FUNCTION_BLOCK FB_SFP_EGU_EGK_IO_Link_Cyclic_Protocol

   VAR_INPUT 
	  	  	
	  b_RELEASE_FUNKTION_BLOCK : BOOL; 
      b_00_FAST_STOP : BOOL;
      b_01_STOP : Bool;
      b_02_ACKNOLEDGE : Bool;
      b_03_PREPARE_FOR_SHUTDOWN : Bool;
      b_04_SOFTRESET : Bool;
      b_05_RELEASE_FOR_MANUAL_MOVEMENT : BOOL;
      b_06_REPEAT_COMMAND_TOGGLE : Bool;
      b_07_GRIP_DIREKTION : BOOL;
	  
      b_08_JOG_MODE_NEGATIVE : Bool;
      b_09_JOG_MODE_POSITIVE : Bool;
      b_11_RELEASE_WORKPIECE : BOOL;
      b_12_GRIP_WORKPIECE : Bool;
      b_13_MOVE_TO_ABSOLUTE_POS : Bool;
      b_14_MOVE_TO_RELATIVE_POS : Bool;
      b_16_GRIP_WORKPIECE_AT_EXPECTED_POSITION : BOOL;
	  b_31_GRIP_FORCE_AND_POSITION_MAINTAINANCE_ACTIVATED : BOOL; 
      di_POSSITIONING : DInt;
      di_VELOCITY : DInt;
      di_GRIPPING_FORCE : DINT;
	  
	  dw_STATUS_DWORD_GRIPPER : DWORD;
	  di_IN_ACTUAL_POSITION : DINT;
	  dw_IN_DIAGNOSE : DWORD;
   END_VAR

   VAR_OUTPUT 
	  
      b_00_READY_FOR_OPPERATION : Bool;
      b_01_CONTOL_AUTHORITY_FIELDBUS : Bool;
      b_02_READY_FOR_SHUTDOWN : Bool;
      b_03_NOT_FEASIBLE : Bool;
      b_04_COMMAND_SUCCESSFULLY_PROCESSED : Bool;
      b_05_COMMAND_RECEIVED_TOGGLE : Bool;
      b_06_WARNING : Bool;
      b_07_ERROR : Bool;
      b_08_BRAKE_RELEASD : Bool;
      b_09_SOFTWARELIMIT_REACHED : Bool;
      b_10_REFERENCED : Bool;
      b_11_NO_WORKPIECE_DETECTED : Bool;
      b_12_WORKPIECE_GRIPPED : Bool;
      b_13_POSITION_REACHED : Bool;
      b_14_WORKPIECE_PRE_GRIPPED_STARTED : Bool;
      b_16_WORKPIECE_LOST : Bool;
      b_17_WRONG_WORKPIECE_DETECTED : BOOL;
	  b_31_ACTIVATE_GRIP_FORCE_AND_POSITION_MAINTAINANCE : BOOL;
	  di_ACTUAL_POSITION : DINT;
      i_DIAGNOSE_WARNUNG : Word;
      i_DIAGNOSE_ERROR : WORD;
	  
	  dw_CONTROL_DW_GRIPPER : DWORD;
	  di_OUT_POSSITIONING : DINT;
	  di_OUT_VELOCITY : DINT;
	  di_OUT_GRIPPING_FORCE : DINT;
	  
   END_VAR
   
   
   VAR_TEMP 
      b_Temp_OUT_15 : BOOL;
	  b_Temp_OUT_18 : BOOL;
	  b_Temp_OUT_19 : BOOL;
	  b_Temp_OUT_20 : BOOL;
	  b_Temp_OUT_21 : BOOL;
	  b_Temp_OUT_22 : BOOL;
	  b_Temp_OUT_23 : BOOL;
	  b_Temp_OUT_24 : BOOL;
	  b_Temp_OUT_25 : BOOL;
	  b_Temp_OUT_26 : BOOL;
	  b_Temp_OUT_27 : BOOL;
	  b_Temp_OUT_28 : BOOL;
	  b_Temp_OUT_29 : BOOL;
	  b_Temp_OUT_30 : BOOL;
	  
	  b_Temp_IN_1 : BOOL;
	  b_Temp_in_2 : BOOL;
	  b_Temp_in_3 : BOOL;
	  b_Temp_in_4 : BOOL;
	  b_Temp_in_5 : BOOL;
	  b_Temp_in_6 : BOOL;
	  b_Temp_in_7 : BOOL;
	  b_Temp_in_8 : BOOL;
	  b_Temp_in_9 : BOOL;
	  b_Temp_in_10 : BOOL;
	  b_Temp_in_11 : BOOL;
	  b_Temp_in_12 : BOOL;
	  b_Temp_in_13 : BOOL;
	  b_Temp_in_14 : BOOL;
	  b_Temp_in_15 : BOOL;
	  b_Temp_in_16 : BOOL;
	  b_Temp_in_17 : BOOL;
	  b_Temp_in_18 : BOOL;
	  b_Temp_in_19 : BOOL;
	  b_Temp_in_20 : BOOL;
	  b_Temp_in_21 : BOOL;
	  b_Temp_in_22 : BOOL;
	  b_Temp_in_23 : BOOL;
	  b_Temp_in_24 : BOOL;
	  b_Temp_in_25 : BOOL;
	  b_Temp_in_26 : BOOL;
	  b_Temp_in_27 : BOOL;
	  b_Temp_in_28 : BOOL;
	  b_Temp_in_29 : BOOL;
	  b_Temp_in_30 : BOOL;
	  b_Temp_in_31 : BOOL;
	  	  
   END_VAR
(*
   VAR 
	  TYPE Input:
	  STRUCT 
      //Input : Struct
         dw_Status_DW : DWord;
         di_Actual_Position : DInt;
         di_Reserved_byte_4_to_byte_7 : DInt;
         i_Diagnostic_Warning : Word;
         i_Diagnostic_Error : Word;
      END_STRUCT
	  END_TYPE
		  
      TYPE Status_DW:
		  STRUCT
         b_Ready_For_Operation : BOOL;
         b_Control_Authority : Bool;
         b_Ready_For_Shutdown : Bool;
         b_Not_Feasible : Bool;
         b_Success : Bool;
         b_Command_Received_Toggle : Bool;
         b_Warning : Bool;
         b_Error : Bool;
         b_Brake_released : Bool;
         b_Sofwarelimit : Bool;
         b_Referenced : Bool;
         b_No_Workpiece_Detected : Bool;
         b_Gripped : Bool;
         b_Position_Reached : Bool;
         b_Pre_Gripped : Bool;
         b_Reserved_1_6 : Bool;
         b_Workpiece_Lost : Bool;
         b_Wrong_Workpiece_Detected : Bool;
         b_Reserved_2_2 : Bool;
         b_Reserved_2_3 : Bool;
         b_Reserved_2_4 : Bool;
         b_Reserved_2_5 : Bool;
         b_Reserved_2_6 : Bool;
         b_Reserved_2_7 : Bool;
         b_Reserved_3_0 : Bool;
         b_Reserved_3_1 : Bool;
         b_Reserved_3_2 : Bool;
         b_Reserved_3_3 : Bool;
         b_Reserved_3_4 : Bool;
         b_Reserved_3_5 : Bool;
         b_Reserved_3_6 : Bool;
         b_Reserved_3_7 : Bool;
      END_STRUCT
	  END_TYPE
	  
	  TYPE Output:
		  STRUCT
         dw_Steuerwort : DWord;
         di_Position : DInt;
         di_Velocity : DInt;
         di_Gripping_Force : DInt;
      END_STRUCT
	  END_TYPE
	  
	  Control_DW: STRUCT;
		  
	  END_STRUCT
      TYPE Control_DW:
		STRUCT 
         b_Fast_Stop : Bool;
         b_Stop : Bool;
         b_Acknoledge : Bool;
         b_Prerare_For_Shutdown : Bool;
         b_Softreset : Bool;
         b_Release_Brake : Bool;
         b_Repeat_Command_Toggle : Bool;
         b_Grip_Direction : Bool;
         b_Jog_Mode_Negative : Bool;
         b_Jog_Mode_Positive : Bool;
         b_Reference : Bool;
         b_Release_Workpiece : Bool;
         b_Grip_Workpiece : Bool;
         b_Move_To_Absolute_Position : Bool;
         b_Move_To_Relative_Position : Bool;
         b_Reserved_1_7 : Bool;
         b_Grip_Workpiece_With_Expected_Position : Bool;
         b_Reserved_2_1 : Bool;
         b_Reserved_2_2 : Bool;
         b_Reserved_2_3 : Bool;
         b_Reserved_2_4 : Bool;
         b_Reserved_2_5 : Bool;
         b_Reserved_2_6 : Bool;
         b_Reserved_2_7 : Bool;
         b_Reserved_3_0 : Bool;
         b_Reserved_3_1 : Bool;
         b_Reserved_3_2 : Bool;
         b_Reserved_3_3 : Bool;
         b_Reserved_3_4 : Bool;
         b_Reserved_3_5 : Bool;
         b_Reserved_3_6 : Bool;
         b_Reserved_3_7 : Bool;
      END_STRUCT
	  END_TYPE
      //GETIO_Instance {InstructionName := 'GETIO'; LibVersion := '1.1'} : GETIO;
      //SETIO_Instance {InstructionName := 'SETIO'; LibVersion := '1.2'} : SETIO;
   END_VAR

   VAR_TEMP 
      reserved_ed_8 : DInt;
   END_VAR

*)



	(*
	FUNCTION_BLOCK FB_SFP_Zyclic_Protokol
	TITLE = 'FB_SFP_EGU_EGK_IO_Link_Cyclic_Protocol'
	VERSION : '1.0.1'
	AUTHOR  : 'SCHUNK'
	NAME    : 'FB_Zyklische_Kommunikation_SFP_Beckhoff TwinCAT 3'
	FAMILY  : 'SCHUNK'
	Projekt Nr.:
	=============================================================================
	 Schunk GmbH&Co.KG
	 (c)Copyright (2022) All Rights Reserved
	-----------------------------------------------------------------------------
	 Library:       Schunk
	 Tested with:   TWINCAT 3 Build 4024.32
	 Engineering:   TWINCAT 3 Build 4024.32
	 Restrictions:  XXX(OB types, etc.)
	 Requirements:  (hardware, technological package, memory needed, etc.)
	 Functionality: The Funktion Block communicates Cyclic with the Gripper to read and Wright Data
	  
	*************************************************************************
	Historie
	####################
	1.0.1
	- Bugfix Input Bit 31
	
	####################
	1.0.0
	Release Funktion Block
	
	
	*************************************************************************)
	
	//MANUAL ENGLISH 
	    
	    // Statement section REGION
	    
	    (*************************************************************************    
	    The function block is TO read AND transfer cyclic parameters that are changed FOR specific functions in the device
	    can be used TO make The application process safer OR faster.
	    
	    Input parameters:
	    ------------------
	    b_RELEASE_FUNKTION_BLOCK		: Release FOR processing the block
	    
	    b_00_FAST_STOP					: immediate shutdown OF The process currently running in The gripper AND shutdown OF The motor phases
	    b_01_STOP						: Pausing AND stopping the currently running process.
	    b_02_ACKNOLEDGE 				: Acknowledge fault
	    b_03_PREPARE_FOR_SHUTDOWN		: Initiate the restoration OF data on The device in preparation FOR switching off OR rebooting
	    b_04_SOFTRESET					: Warm start OF The device
	    b_05_RELEASE_FOR_MANUAL_MOVEMENT: The brake can be released FOR 5 seconds in the "ERROR_FAST_STOP" state
	    b_06_REPEAT_COMMAND_TOGGLE		: The command that is still pending can, IF it is a repeatable command, be repeated without loss OF Time FOR each positive AND negative change OF this bit
	    b_07_GRIP_DIRECTION				: determines The gripping direction. FALSE = external gripping (the workpiece is gripped from the outside) / True = internal gripping (the workpiece is gripped from the inside).
	    
	    b_08_JOG_MODE_NEGATIVE			: Simple movement OF The device in negative direction. Function also possible without "REFERENCE".
	    b_09_JOG_MODE_POSITIVE			: Simple movement OF The device in The positive direction. Function also possible without "REFERENCE".
	    b_10_Reserved					: 
	    b_11_RELEASE_WORKPIECE			: IF The status is "GRIPPED", the gripper is opened in the opposite direction AND the workpiece is released
	    b_12_GRIP_WORKPIECE				: the gripper executes a movement that should lead TO gripping a workpiece. Internal speed parameters are used here
	    b_13_MOVE_TO_ABSOLUTE_POSITION	: The gripper jaws are moved TO The position specified in The cyclic protocol at The specified speed.
	    b_14_MOVE_TO_RELATIVE_POSITION	: The gripper jaws are moved TO The calculated position with The position specified in The cyclic protocol at The specified speed.
	    b_15_Reserved					: 
		
	    b_16_GRIP_WORKPIECE_AT_EXPECTED_POSITION : the gripper performs a movement which is intended to grip a workpiece. Here, the position value is assumed as the workpiece size. Due to the workpiece size, it is pre-positioned accordingly and then gripped. See software manual for more information.
		b_17_Reserved					: 
		b_18_Reserved					: 
		b_19_Reserved					: 
		b_20_Reserved					: 
		b_21_Reserved					: 
		b_22_Reserved					: 
		b_23_Reserved					: 
		
		b_24_Reserved					: 
		b_25_Reserved					: 
		b_26_Reserved					: 
		b_27_Reserved					: 
		b_28_Reserved					: 
		b_29_Reserved					: 
		b_30_Reserved					: 
		b_31_ACTIVATE_GRIP_FORCE_AND_POSITION_MAINTAINANCE	: Maintaining the gripping force by locking the gripper jaws with a brake.
	    
		dw_STATUS_DWORD_GRIPPER 		: Input double word of the gripper which comes from the hardware and is split into individual bits in the block
		di_IN_ACTUAL_POSITION 			: Current position of the gripper. Is only passed on to the output parameter of the block.
		dw_IN_DIAGNOSE 					: Diagnostic double word of the gripper. Is split into warning and error in the block.
		
	    #################
	    
	    Output parameters:
	    ------------------
	    
	    b_00_READY_FOR_OPPERATION		:   indicates that the gripper is ready FOR operation
	    b_01_CONTOL_AUTHORITY_FIELDBUS  :   indicates whether the fieldbus has control authority over the gripper
	    b_02_READY_FOR_SHUTDOWN			:   signals readiness FOR shutdown OR restart after the request "Prepare for shutdown"
	    b_03_NOT_FEASIBLE				:	Indicates that the last issued command cannot be executed.
	    									Possible causes are:
	        								- a new command was sent although the command that is still active has NOT yet been processed.
	        								- 2 OR more control commands simultaneously active in the control word
	        								- Parameter data FOR position, speed OR force are outside the permissible limits.
	    
	    b_04_COMMAND_SUCCESSFULLY_PROCESSED	: indicates that the last executable command was successfully processed.
	    b_05_COMMAND_RECEIVED_TOGGLE		: Indicates that a command was sent TO The gripper via The bus. the command does NOT have TO be processed OR started at the time it is displayed.
	    b_06_WARNING						: signals a warning in the gripper, e.g. temperature warning
	    b_07_ERROR							: signals a fault in the gripper, e.g. rapid stop
		
	    b_08_BRAKE_RELEASD					: Signals that the brake is released IF a brake is installed in The gripper.
	    b_09_SOFTWARELIMIT_REACHED			: indicates that the gripper has reached a software limit
	    b_10_REFERENCED						: indicates that the gripper is referenced
	    b_11_NO_WORKPIECE_DETECTED			: indicates that no workpiece was detected
	    b_12_WORKPIECE_GRIPPED				: signals that a workpiece has been gripped
	    b_13_POSITION_REACHED				: signals that the relative OR absolute position has been approached
	    b_14_WORKPIECE_PRE_GRIPPED_STARTED  : indicates that the gripper has started the pre-gripping function
		b_15_Reserved						: 
		
	    b_16_WORKPIECE_LOST					: signals that the gripped workpiece was lost
	    b_17_WRONG_WORKPIECE_DETECTED		: signals that a wrong workpiece was detected
		b_18_RESERVED						: 
		b_19_RESERVED						: 
		b_20_RESERVED						: 
		b_21_RESERVED						: 
		b_22_RESERVED						: 
		b_23_RESERVED						: 
		
		b_24_RESERVED						: 
		b_25_RESERVED						: 
		b_26_RESERVED						: 
		b_27_RESERVED						: 
		b_28_RESERVED						: 
		b_29_RESERVED						: 
		b_30_RESERVED						: 
		b_31_GRIP_FORCE_AND_POSITION_MAINTAINANCE_ACTIVATED : Maintaining the gripping force by locking the gripper jaws with a brake is active.
		
	    di_ACTUAL_POSITION					: the current position OF The gripper is returned here
	    i_DIAGNOSE_WARNUNG					: Output of the gripper's warning code
	    i_DIAGNOSE_ERROR					: Output of the error code of the gripper
	        
	    *************************************************************************)
	    
// MANUAL GERMAN
	    
	(*************************************************************************
	    Der Baustein soll Zyklische Parameter einlesen und übertragen, welche für bestimmte Funktionen im Gerät geändert 
	    werden können um den Applikationsprozess sicherer oder schneller zu machen.
	    
	    Eingangsparameter:
	    ------------------
	    
	    b_RELEASE_FUNKTION_BLOCK : Freigabe zur Bearbeitung des Bausteins
	    
	    b_00_FAST_STOP					: sofortiges Abschalten des aktuell im Greifer laufenden Prozesses und abschalten der Motorphasen
	    b_01_STOP						: Anhalten und Stoppen des Aktuell laufenden Prozesses.
	    b_02_ACKNOLEDGE					: Störung Quittieren
	    b_03_PREPARE_FOR_SHUTDOWN		: Anstoßen der Rückspeicherung von Daten auf dem Grät un Vorbereitung zum Ausschalten oder Reboot
	    b_04_SOFTRESET					: Warmstart des Gerätes
	    b_05_RELEASE_FOR_MANUAL_MOVEMENT: Lösen der Bremse für 5 Sekunden im Zustand "ERROR_FAST_STOP" möglich
	    b_06_REPEAT_COMMAND_TOGGLE		: Das Noch anstehende Kommando kann, sofern es ein wiederholbares Kommando ist, ohne zeitverlust bei jedem positiven und negativen wechsel dieses Bits wiederholt werden 
	    b_07_GRIP_DIRECTION				: legt die Greifrichtung fest. FALSE = Ausengreifen (Das Werkstück wird von ausen gegriffen) / True = Innengreifen (Das Werkstück wird von innen gegriffen). 
	    
	    b_08_JOG_MODE_NEGATIVE			: einfaches Verfahren des Gerätes in negative Richtung. Funktion auch ohne Referenz möglich.
	    b_09_JOG_MODE_POSITIVE			: einfaches Verfahren des Gerätes in positive Richtung. Funktion auch ohne Referenz möglich.
	    b_10_RESERVED					: Referenzieren des Gerätes wird angestoßen
	    b_11_RELEASE_WORKPIECE			: Bei Status "GRIPPED" wird der Greifer in die entgegegesetzte Richtung geöffnet und das Werkstück freigegeben
	    b_12_GRIP_WORKPIECE				: der Greifer führt eine Bewegung aus, welche zum greifen eines Werkstückes führen soll. Hierbei werden interne Geschwindigkeitsparameter genommen
	    b_13_MOVE_TO_ABSOLUTE_POSITION	: Die Greiferbacken werden auf die im Zyklischen Protokoll vorgegebene Position mit der vorgegebenen Geschwindigkeit gefahren. 
	    b_14_MOVE_TO_RELATIVE_POSITION	: Die Greiferbacken werden auf die errechnete Position mit der im Zyklischen Protokoll vorgegebene Position mit der vorgegebenen Geschwindigkeit gefahren.
	    b_15_Reserved					: 
		
	    b_16_GRIP_WORKPIECE_AT_EXPECTED_POSITION : der Greifer führt eine Bewegung aus, welche zum greifen eines Werkstückes führen soll. Hirbei wird der Positionswert als Werkstückgröße angenommen. aufgrund der Werkstückgröße wird entsprechend Vorpositioniert und dann gegriffen. Weitere Informationen siehe Softwarehandbuch.
		b_17_Reserved					: 
		b_18_Reserved					: 
		b_19_Reserved					: 
		b_20_Reserved					: 
		b_21_Reserved					: 
		b_22_Reserved					: 
		b_23_Reserved					: 
		
		b_24_Reserved					: 
		b_25_Reserved					: 
		b_26_Reserved					: 
		b_27_Reserved					: 
		b_28_Reserved					: 
		b_29_Reserved					: 
		b_30_Reserved					: 
		b_31_ACTIVATE_GRIP_FORCE_AND_POSITION_MAINTAINANCE	: Erhaltung der Greifkraft durch festsetzen der Greifbackendurch eine Bremse.
              

		dw_STATUS_DWORD_GRIPPER 		: Eingangsdoppelwort des Greifers welches von der Hardware kommt und im Baustein in einzelbits aufgesplittet wird
		di_IN_ACTUAL_POSITION 			: Aktuelle Position des Greifers. Wird nur durchgereicht auf den Ausgangsparameter des Bausteins.
		dw_IN_DIAGNOSE 					: Diagnosedoppelwort des Greifers. Wird im Baustein zu Warning und Error aufgesplittet.
            
	    ##################    
    
	    Ausgangsparameter:
	    ------------------
	    
	    b_00_READY_FOR_OPPERATION			: zeigt die Betriebsbereitschaft des Greifers an
	    b_01_CONTOL_AUTHORITY_FIELDBUS		: zeigt an, ob der Feldbus die Steuerhoheit über den Greifer hat
	    b_02_READY_FOR_SHUTDOWN				: signalisiert die Bereitschaft zum Abschalten bzw Neustarten nach der Anforderung "Prepare for shutdown"
	    b_03_NOT_FEASIBLE					: Zeigt an, das der zuletzt abgesetzte Befehl nicht ausgeführt werden kann.
	                            				Mögliche Ursachen sind:
	                                			- ein neuer Befehl wurde abgesetzt, obwohl der noch aktive Befehl noch nicht abgearbeitet wurde.
	                                			- 2 oder mehr Steuerbefehle gleichzeitig aktiv im Steuerwort
	                                			- Parameterdaten von Position, Geschwindigkeit oder Kraft liegen auserhalb der Zulässigen grenzen. 
	                                
	    b_04_COMMAND_SUCCESSFULLY_PROCESSED	: zeigt das erfolgreiche Abarbeiten des letzten ausführbaren Befehls an.
	    b_05_COMMAND_RECEIVED_TOGGLE		: Zeigt an, das ein Befehl über den Bus an den Greufer gesendet wurde. zum Zeitpunkt der Anzeige muß der Befehl noch nicht abgearbeitet oder gestartet sein.
	    b_06_WARNING						: signalisiert eine Warnung im Greifer, z.B. Temperaturwarnung
	    b_07_ERROR							: signalisiert eine Störung im Greifer, z.B. Schnellstop
		
	    b_08_BRAKE_RELEASD					: Signalisiert, dass die Bremse geöffnet ist, sofern eine Bremse im Greifer verbaut ist.
	    b_09_SOFTWARELIMIT_REACHED			: signalisiert, das der Greifer eine Softwarelimit angefahren hat
	    b_10_REFERENCED						: signalisiert, das der Greifer referenziert ist 
	    b_11_NO_WORKPIECE_DETECTED			: signalisiert, dass kein Werkstück erkannt wurde
	    b_12_WORKPIECE_GRIPPED				: signalisiert, dass ein Werkstück gegriffen wurde
	    b_13_POSITION_REACHED				: signalisiert, dass die relative oder absolute Possition angefahren wurde
	    b_14_WORKPIECE_PRE_GRIPPED_STARTED  : signalisiert, dass der Greifer die Pre Gripping Funktion angestoßen hat
		b_15_RESERVED						: 
		
	    b_16_WORKPIECE_LOST					: signalisiert, dass das gegriffene Werkstück verloren ging
	    b_17_WRONG_WORKPIECE_DETECTED		: signalisiert, das ein falsches Werkstück erkannt wurde
		b_18_RESERVED						: 
		b_19_RESERVED						: 
		b_20_RESERVED						: 
		b_21_RESERVED						: 
		b_22_RESERVED						: 
		b_23_RESERVED						: 
		
		b_24_RESERVED						: 
		b_25_RESERVED						: 
		b_26_RESERVED						: 
		b_27_RESERVED						: 
		b_28_RESERVED						: 
		b_29_RESERVED						: 
		b_30_RESERVED						: 
		b_31_GRIP_FORCE_AND_POSITION_MAINTAINANCE_ACTIVATED : Erhaltung der Greifkraft durch festsetzen der Greifbackendurch eine Bremse ist aktiv.
				
	    di_ACTUAL_POSITION					: hier wird die aktuelle Possition des Greifers zurückgegeben
	    i_DIAGNOSE_WARNUNG					: Ausgabe des Warnungscodes des Greifers
	    i_DIAGNOSE_ERROR					: Ausgabe des Störungscodes des Greifers
	    
	*************************************************************************)
	    
	// Release FB
	    // Statement section REGION
	    		
	    IF  
				b_RELEASE_FUNKTION_BLOCK = TRUE
	    THEN
	       
			b_00_READY_FOR_OPPERATION 			:= DW_STATUS_DWORD_GRIPPER.0;
			b_01_CONTOL_AUTHORITY_FIELDBUS 		:= DW_STATUS_DWORD_GRIPPER.1;
			b_02_READY_FOR_SHUTDOWN 			:= DW_STATUS_DWORD_GRIPPER.2;
			b_03_NOT_FEASIBLE 					:= DW_STATUS_DWORD_GRIPPER.3;
			b_04_COMMAND_SUCCESSFULLY_PROCESSED := DW_STATUS_DWORD_GRIPPER.4;
			b_05_COMMAND_RECEIVED_TOGGLE 		:= DW_STATUS_DWORD_GRIPPER.5;
			b_06_WARNING 						:= DW_STATUS_DWORD_GRIPPER.6;
			b_07_ERROR 							:= DW_STATUS_DWORD_GRIPPER.7;
			b_08_BRAKE_RELEASD 					:= DW_STATUS_DWORD_GRIPPER.8;
			b_09_SOFTWARELIMIT_REACHED 			:= DW_STATUS_DWORD_GRIPPER.9;
			b_10_REFERENCED 					:= DW_STATUS_DWORD_GRIPPER.10;
			b_11_NO_WORKPIECE_DETECTED 			:= DW_STATUS_DWORD_GRIPPER.11;
			b_12_WORKPIECE_GRIPPED 				:= DW_STATUS_DWORD_GRIPPER.12;
			b_13_POSITION_REACHED 				:= DW_STATUS_DWORD_GRIPPER.13;
			b_14_WORKPIECE_PRE_GRIPPED_STARTED 	:= DW_STATUS_DWORD_GRIPPER.14;
			b_Temp_OUT_15 						:= DW_STATUS_DWORD_GRIPPER.15; 
			b_16_WORKPIECE_LOST 				:= DW_STATUS_DWORD_GRIPPER.16;
			b_17_WRONG_WORKPIECE_DETECTED 		:= DW_STATUS_DWORD_GRIPPER.17;
			b_Temp_OUT_18 						:= DW_STATUS_DWORD_GRIPPER.18;
			b_Temp_OUT_19 						:= DW_STATUS_DWORD_GRIPPER.19;
			b_Temp_OUT_20 						:= DW_STATUS_DWORD_GRIPPER.20;
			b_Temp_OUT_21 						:= DW_STATUS_DWORD_GRIPPER.21;
			b_Temp_OUT_22 						:= DW_STATUS_DWORD_GRIPPER.22;
			b_Temp_OUT_23 						:= DW_STATUS_DWORD_GRIPPER.23;
			b_Temp_OUT_24 						:= DW_STATUS_DWORD_GRIPPER.24; 
			b_Temp_OUT_25 						:= DW_STATUS_DWORD_GRIPPER.25; 
			b_Temp_OUT_26 						:= DW_STATUS_DWORD_GRIPPER.26; 
			b_Temp_OUT_27 						:= DW_STATUS_DWORD_GRIPPER.27; 
			b_Temp_OUT_28 						:= DW_STATUS_DWORD_GRIPPER.28; 
			b_Temp_OUT_29 						:= DW_STATUS_DWORD_GRIPPER.29; 
			b_Temp_OUT_30 						:= DW_STATUS_DWORD_GRIPPER.30; 
			b_31_GRIP_FORCE_AND_POSITION_MAINTAINANCE_ACTIVATED := DW_STATUS_DWORD_GRIPPER.31; 
			
			di_ACTUAL_POSITION 					:= di_IN_ACTUAL_POSITION;
			i_DIAGNOSE_WARNUNG 					:= DWORD_TO_WORD(dw_IN_DIAGNOSE);
			i_DIAGNOSE_ERROR 					:= DWORD_TO_WORD(SHR(dw_IN_DIAGNOSE, 16));

 
			dw_CONTROL_DW_GRIPPER.0 := b_00_FAST_STOP;
			dw_CONTROL_DW_GRIPPER.1 := b_01_STOP;
			dw_CONTROL_DW_GRIPPER.2 := b_02_ACKNOLEDGE;
			dw_CONTROL_DW_GRIPPER.3 := b_03_PREPARE_FOR_SHUTDOWN;
			dw_CONTROL_DW_GRIPPER.4 := b_04_SOFTRESET;
			dw_CONTROL_DW_GRIPPER.5 := b_05_RELEASE_FOR_MANUAL_MOVEMENT;
			dw_CONTROL_DW_GRIPPER.6 := b_06_REPEAT_COMMAND_TOGGLE;
			dw_CONTROL_DW_GRIPPER.7 := b_07_GRIP_DIREKTION;
			dw_CONTROL_DW_GRIPPER.8 := b_08_JOG_MODE_NEGATIVE;
			dw_CONTROL_DW_GRIPPER.9 := b_09_JOG_MODE_POSITIVE;
			dw_CONTROL_DW_GRIPPER.10 := b_10_REFERENCED;
			dw_CONTROL_DW_GRIPPER.11 := b_11_RELEASE_WORKPIECE;
			dw_CONTROL_DW_GRIPPER.12 := b_12_GRIP_WORKPIECE;
			dw_CONTROL_DW_GRIPPER.13 := b_13_MOVE_TO_ABSOLUTE_POS;
			dw_CONTROL_DW_GRIPPER.14 := b_14_MOVE_TO_RELATIVE_POS;
			dw_CONTROL_DW_GRIPPER.15 := FALSE;
			dw_CONTROL_DW_GRIPPER.16 := b_16_GRIP_WORKPIECE_AT_EXPECTED_POSITION;
			dw_CONTROL_DW_GRIPPER.17 := FALSE;
			dw_CONTROL_DW_GRIPPER.18 := FALSE;
			dw_CONTROL_DW_GRIPPER.19 := FALSE;
			dw_CONTROL_DW_GRIPPER.20 := FALSE;
			dw_CONTROL_DW_GRIPPER.21 := FALSE;
			dw_CONTROL_DW_GRIPPER.22 := FALSE;
			dw_CONTROL_DW_GRIPPER.23 := FALSE;
			dw_CONTROL_DW_GRIPPER.24 := FALSE;
			dw_CONTROL_DW_GRIPPER.25 := FALSE;
			dw_CONTROL_DW_GRIPPER.26 := FALSE;
			dw_CONTROL_DW_GRIPPER.27 := FALSE;
			dw_CONTROL_DW_GRIPPER.28 := FALSE;
			dw_CONTROL_DW_GRIPPER.29 := FALSE;
			dw_CONTROL_DW_GRIPPER.30 := FALSE;
			dw_CONTROL_DW_GRIPPER.31 := b_31_ACTIVATE_GRIP_FORCE_AND_POSITION_MAINTAINANCE;

			di_OUT_POSSITIONING 	:= di_POSSITIONING;
			di_OUT_VELOCITY 		:= di_VELOCITY;
			di_OUT_GRIPPING_FORCE 	:= di_GRIPPING_FORCE;
			
	    END_IF;

END_FUNCTION_BLOCK
